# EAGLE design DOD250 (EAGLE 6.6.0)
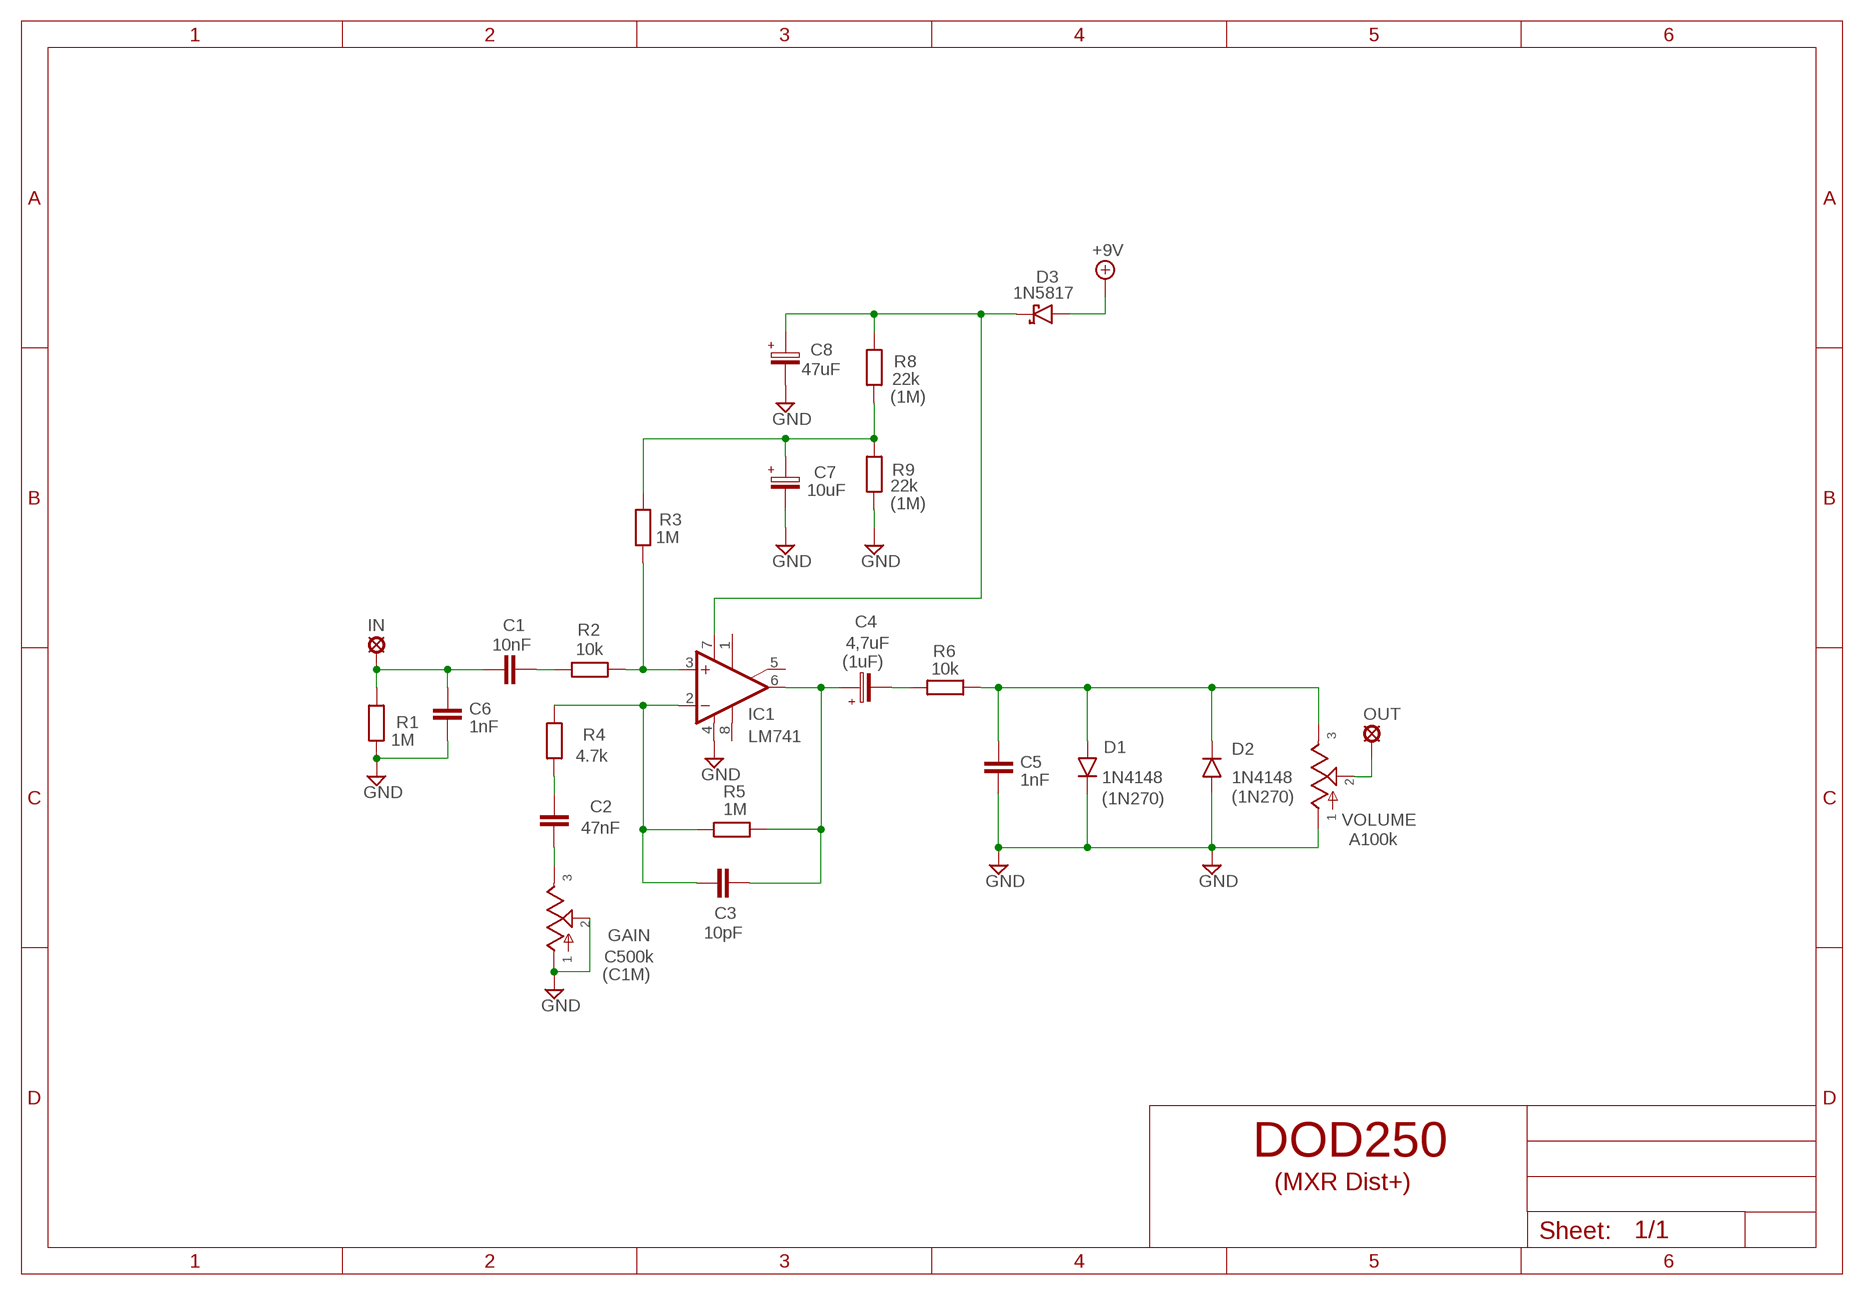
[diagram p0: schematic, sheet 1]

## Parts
+9V  +9V  +9V(T)1  [ROUND]
C1  10nF  1NF-15NF  [3,5MM]
C2  47nF  10NF-47NF"  [4,5MM]
C3  10pF  050X030_0252  [050X030_025_2]
C4  4,7uF  063-EU2  [063_025_2]
C5  1nF  1NF-6,8NF  [3,5MM]
C6  1nF  1NF-6,8NF  [3,5MM]
C7  10uF  063-EU  [063_025]
C8  47uF  063-EU  [063_025]
D1  1N4148  DO07  [DO07]
D2  1N4148  DO07  [DO07]
D3  1N5817  [DO41-3]
GAIN  C500k  POT16MM  [16MM]
GND  GND  GND(T)1  [ROUND]
GND6  GND  GND(T)1  [ROUND]
IC1  LM741  [TO99]
IN  MCS10B  [MCS10B]
OUT  MCS10B  [MCS10B]
R1  1M  6MM-EU3  [R0207/3]
R2  10k  6MM-EU3  [R0207/3]
R3  1M  6MM-EU3  [R0207/3]
R4  4.7k  6MM-EU3  [R0207/3]
R5  1M  6MM-EU3  [R0207/3]
R6  10k  6MM-EU3  [R0207/3]
R8  22k  6MM-EU3  [R0207/3]
R9  22k  6MM-EU3  [R0207/3]
VOLUME  A100k  POT16MM  [16MM]

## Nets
+9V: +9V.1(+9V) D3.A
GND: C5.2 C6.2 C7.- C8.- D1.C D2.A GAIN.1 GAIN.2 GND6.1(GND) GND.1(GND) IC1.4(V-) R1.1 R9.1 VOLUME.1
N$1: C2.2 GAIN.3
N$2: C4.- R6.1
N$3: C7.+ R3.2 R8.1 R9.2
N$4: OUT.MP VOLUME.2
N$5: C1.2 R2.1
N$6: IC1.3(+IN) R2.2 R3.1
N$7: C3.2 C4.+ IC1.6(OUT) R5.2
N$8: C5.1 D1.A D2.C R6.2 VOLUME.3
N$9: C3.1 IC1.2(-IN) R4.2 R5.1
N$10: C2.1 R4.1
N$11: C1.1 C6.1 IN.MP R1.2
N$18: C8.+ D3.C IC1.7(V+) R8.2
Unconnected: IC1.1(ON1) IC1.5(ON2) IC1.8(OPT)

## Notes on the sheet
- (1M)
- (1M)
- (1uF)
- (1N270) | (1N270)
- (C1M)
- (MXR Dist+)

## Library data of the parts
+9V = gm-supply:+9V(T): +9V Voltage Supply
C1 = Mylar Kondensaattorit:1NF-15NF: 1nF-15nF
C2 = Mylar Kondensaattorit:10NF-47NF: 10nF-47nF
C3 = Keraamiset kondensaattorit:050X030_025: 47 - 120pF
C4 C7 C8 = Elektrolyytit:063-EU
C5 C6 = Mylar Kondensaattorit:1NF-6,8NF: 1nF-6,8nF
D1 D2 = Diodit:DO07: DO-07 Package
D3 = Diodit:1N5817
GAIN VOLUME = gm-pots:POT: Potentiometers the arrow indicates the clockwise motion of th wiper (lug 2) fully counter clockwise there is no resistance between lugs 1 and 2 fully clockwise the resistance between lugs 1 and 2 is the value of the pot
GND GND6 = gm-supply:GND(T): Ground
IC1 = Operaatiovahvistimet:*741: OP AMP
IN OUT = Padit:MCS10B: SOLDER PAD
R1-R6 R8 R9 = Vastukset:6MM-EU: 6mm Resistors (European schematic symbol)

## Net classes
0 default: width 0.406 mm

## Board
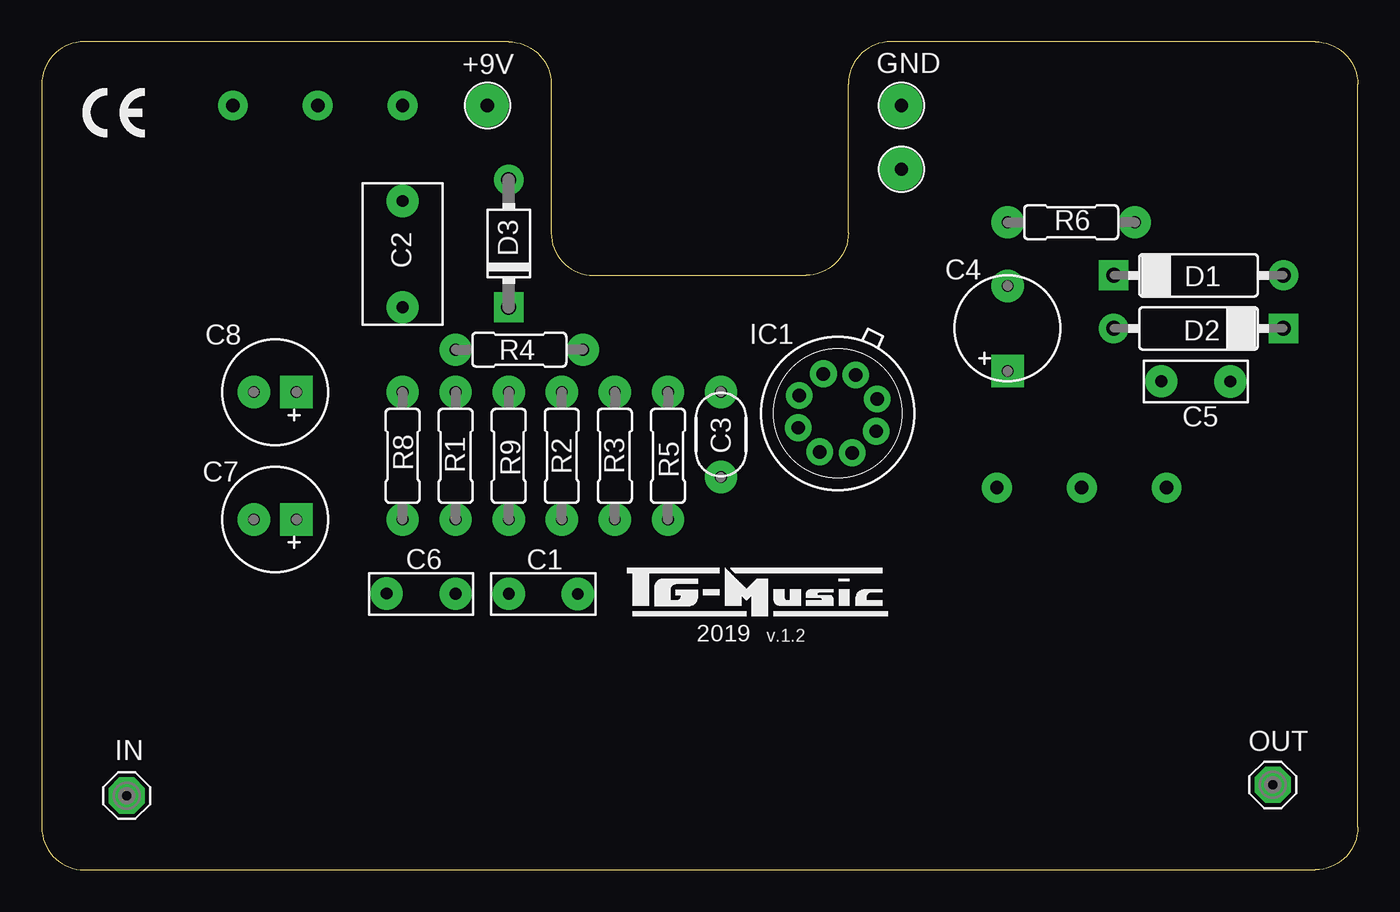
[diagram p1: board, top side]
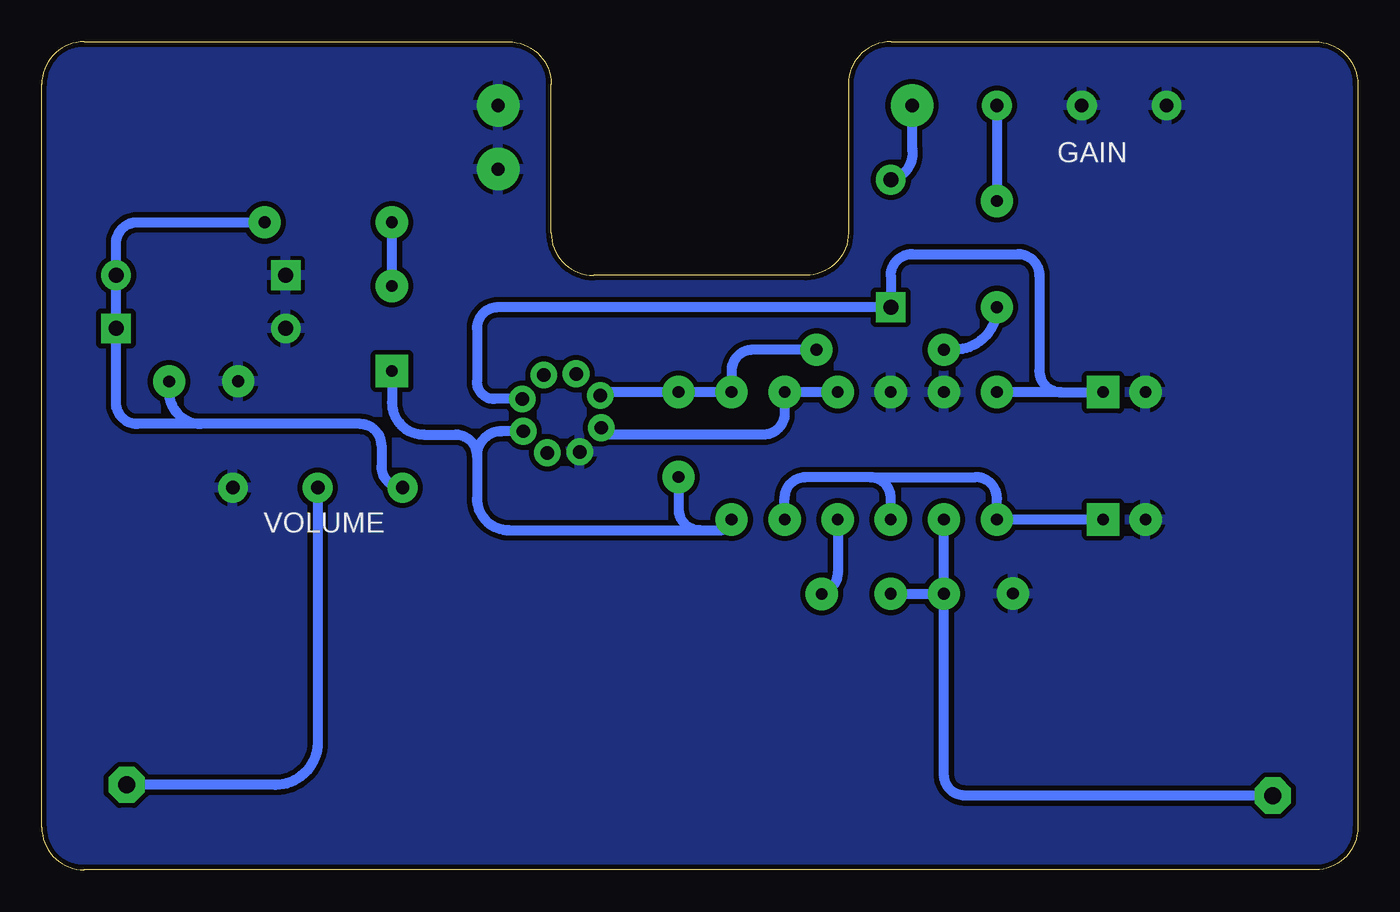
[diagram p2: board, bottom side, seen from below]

Size 78.74 x 49.53 mm. Coordinates in mm from the lower left corner, seen from the top.
Outline: 7.62,49.53 3.81,49.53
Outline: 78.74,2.54 78.74,46.99 arc90 76.2,49.53 50.8,49.53 arc90 48.26,46.99 48.26,38.1 arc-90 45.72,35.56 33.02,35.56 arc-90 30.48,38.1 30.48,46.99 arc90 27.94,49.53 2.54,49.53 arc90 0,46.99 0,2.54 arc90 2.54,0 76.2,0 arc90 78.74,2.54
Copper layers (1*16): Top 0.035mm / dielectric 1.5mm / Bottom 0.035mm
Design rules "ITEADstudio": minimum track width 10mil, minimum drill 12mil, track to track 12mil, track to pad 12mil, pad to pad 12mil, via to via 12mil, smd to smd 0mil, copper to edge 12mil, drill to drill 12mil, minimum pad ring 10mil, minimum via ring 6mil, stop-mask expansion 4mil, vias tented up to drill 100mil, thermal gap 10mil

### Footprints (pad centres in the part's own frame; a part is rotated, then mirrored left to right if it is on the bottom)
ROUND = drill 0.8 pad 2.54: 1 0,0
3,5MM = drill 0.7 pad 1.93: 1 -1.905,0; 2 2.221,-0.016
4,5MM = drill 0.7 pad 1.93: 1 -3.175,0; 2 3.175,0
050X030_025_2 = drill 0.7 pad 1.93: 1 -2.54,0; 2 2.54,0
063_025_2 = drill 0.7 pad 1.93 square: + -2.54,0 | drill 0.7 pad 1.93: - 2.54,0
063_025 = drill 0.7 pad 1.93 square: + -1.27,0 | drill 0.7 pad 1.93: - 1.27,0
DO07 = drill 0.9 pad 1.778: A 5.08,0 | drill 0.9 pad 1.778 square: C -5.08,0
DO41-3 = drill 0.9 pad 1.778: A 3.81,0 | drill 0.9 pad 1.778 square: C -3.81,0
16MM = drill 0.8 pad 1.778: 1 5.08,0; 2 0,0; 3 -5.08,0
TO99 = drill 0.8 pad 1.6: 1 -1.778,-1.778; 2 0,-2.54; 3 1.778,-1.778; 4 2.54,0; 5 1.778,1.778; 6 0,2.54; 7 -1.778,1.778; 8 -2.54,0
MCS10B = drill 1.016 pad 2.159 octagon: MP 0,0
R0207/3 = drill 0.7 pad 1.93: 1 -3.81,0; 2 3.81,0

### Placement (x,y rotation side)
+9V  26.67,45.72 0 top
C1  29.84,16.51 0 top
C2  21.59,36.83 90 top
C3  40.64,26.04 270 top
C4  57.78,32.38 90 top
C5  69.22,29.21 180 top
C6  22.86,16.51 180 top
C7  13.97,20.95 180 top
C8  13.97,28.57 180 top
D1  69.22,35.56 0 top
D2  69.22,32.38 180 top
D3  27.94,37.47 90 top
GAIN  16.51,45.72 180 top
GND  51.44,45.72 0 top
GND6  51.44,41.91 0 top
IC1  47.62,27.3 245 top
IN  5.08,4.45 0 top
OUT  73.66,5.08 0 top
R1  24.77,24.77 270 top
R2  31.11,24.77 90 top
R3  34.29,24.77 270 top
R4  28.57,31.11 0 top
R5  37.47,24.77 270 top
R6  61.59,38.73 0 top
R8  21.59,24.77 90 top
R9  27.94,24.77 270 top
VOLUME  62.23,22.86 0 top

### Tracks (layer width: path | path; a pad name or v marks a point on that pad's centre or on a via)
+9V
  Bottom 0.61: +9V.1 26.67,43.18 arc90 D3.A
GND
  pour Bottom: 0,1.91 0,46.99 arc-90 2.54,49.53 27.94,49.53 arc-90 30.48,46.99 30.48,38.1 arc90 33.02,35.56 45.72,35.56 arc90 48.26,38.1 48.26,46.99 arc-90 50.8,49.53 76.2,49.53 arc-90 78.74,46.99 78.74,2.54 arc-90 76.2,0 1.91,0 arc-90
N$1
  Bottom 0.61: GAIN.3 C2.2
N$2
  Bottom 0.61: C4.- R6.1
N$3
  Bottom 0.61: R3.2 34.29,22.23 arc90 33.02,23.5 29.21,23.5 | 29.21,23.5 22.86,23.5 arc90 21.59,22.23 R8.1 C7.+ | R9.2 27.94,22.23 arc-90 29.21,23.5
N$4
  Bottom 0.61: VOLUME.2 62.23,7.62 arc90 64.77,5.08 OUT.MP
N$5
  Bottom 0.61: R2.1 31.11,17.78 arc90 32.38,16.51 C1.2
N$6
  Bottom 0.61: R2.2 R3.1 34.29,27.3 arc90 35.56,26.04 44.85,26.04 arc90 IC1.3
N$7
  Bottom 0.61: IC1.6 51.24,26.23 arc-90 52.7,24.77 | 52.7,24.77 52.7,22.23 arc-90 50.8,20.32 39.37,20.32 | 39.37,20.32 38.1,20.32 arc-90 R5.2 | C3.2 40.64,21.59 arc-90 39.37,20.32 | C4.+ 57.78,27.94 arc-90 55.88,26.04 53.98,26.04 arc90 52.7,24.77
N$8
  Bottom 0.61: VOLUME.3 arc90 58.42,24.13 58.42,25.4 arc-90 59.69,26.67 69.22,26.67 | 69.22,26.67 73.03,26.67 arc90 74.3,27.94 D2.C D1.A 74.3,37.47 arc90 73.03,38.73 71.12,38.73 R6.2 | C5.1 71.12,28.57 arc-90 69.22,26.67
N$9
  Bottom 0.61: R4.2 36.2,31.11 arc-90 37.47,29.84 R5.1 C3.1 45.13,28.57 arc-90 IC1.2
N$10
  Bottom 0.61: C2.1 arc90 24.13,31.11 R4.1
N$11
  Bottom 0.61: C1.1 C6.1 | C6.1 R1.2 | IN.MP 23.5,4.45 arc90 24.77,5.71 C6.1
N$18
  Bottom 0.61: IC1.7 51.66,28.16 arc90 52.7,29.21 52.7,32.38 arc90 51.44,33.66 D3.C 27.94,35.56 arc90 26.67,36.83 20.32,36.83 arc90 19.05,35.56 19.05,29.84 arc-90 17.78,28.57 | 17.78,28.57 C8.+ | 17.78,28.57 R8.2

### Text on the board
tNames: 2019 | v.1.2
tValues: OUT | +9V | GND | IN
